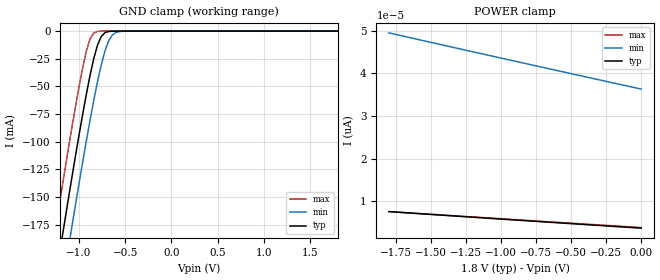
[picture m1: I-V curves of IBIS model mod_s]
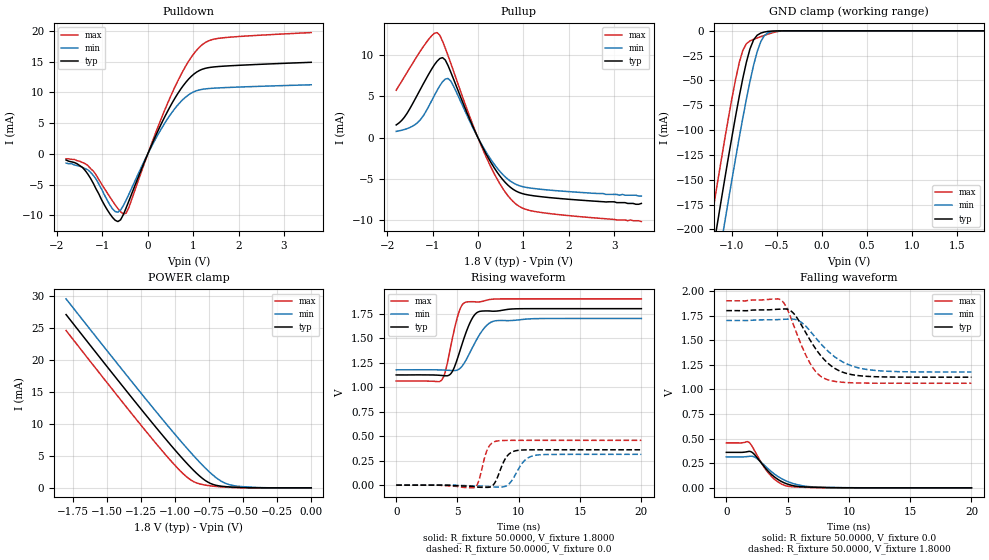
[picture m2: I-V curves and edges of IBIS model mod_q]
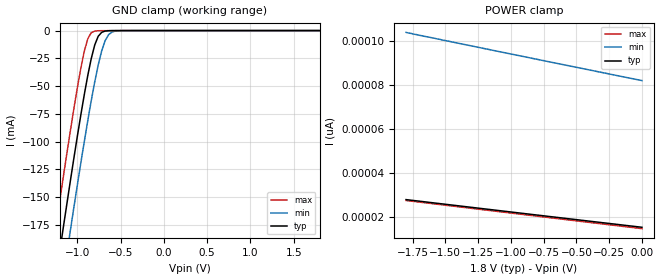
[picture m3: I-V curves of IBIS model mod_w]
| IBIS (I/O, Buffer, Information, Specification) Model, officially
| electronic behavioral standard for Buffer structures of digital pins.
[IBIS ver]  4.0
[File name] m95xxx_tssop8_1d8v.ibs
[File Rev]  16
[Date]  13 December 2012
[Notes]
  (Note1)  This IBIS model includes the TSSOP8 package parasitic data
  (Note2)  This IBIS model considers: VCC= 1.80(TYP), 1.70(MIN), 1.90(MAX)
  (Note3)  This IBIS model has some Notes about the non-monotonicity
   of the I-V curves, but they are not indicative of problems
   inside the model;
[Copyright] (c) 2012 STMicroelectronics
| - M95xxx EEPROM (F8H/P2 process)
| - Voltage Supply Range: 1.7V/1.9V
| - Package: TSSOP8
[Component] M95XXX
[Manufacturer] STMicroelectronics
[Package]
| variable   typ   min   max
R_pkg   0.0   0.0   0.0
L_pkg   0.0H   0.0H   0.0H
C_pkg   0.0F   0.0F   0.0F
[Pin]   signal_name   model_name   R_pin   L_pin   C_pin
1   SN   mod_s   NA   NA   NA
2   Q   mod_q   NA   NA   NA
3   WN   mod_w   NA   NA   NA
4   GND   GND   NA   NA   NA
5   D   mod_s   NA   NA   NA
6   C   mod_s   NA   NA   NA
7   HOLDN   mod_h   NA   NA   NA
8   VCC   POWER   NA   NA   NA
[Package Model]  182696_TSSOP8
[Define Package Model]  182696_TSSOP8
[Manufacturer]  STMicroelectronics
[OEM]  STMicroelectronics
[Description]  8 pin TSSOP package
[Number Of Pins]  8
[Pin Numbers]
|Pin Num   Terminal Name
1   | net1
2   | net2
3   | net3
4   | net4_GND
5   | net5
6   | net6
7   | net7
8   | net8_VDD
[Model Data]
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[End Model Data]
[End Package Model]
| Models and submodels in the file (4): mod_s (Input), mod_q (I/O), mod_w (Input), mod_h (Input)
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|   Model mod_s
[Model]   mod_s   | associated to PIN1 (S), PIN5 (D), PIN6 (CK)
Model_type Input
Vinl   =   0.45V
Vinh   =   1.35V
C_comp   2.119pF   2.023pF   2.433pF
[Temperature Range]   25.0000   85.0000   -40.0000
[Voltage Range]   1.8000V   1.7000V   1.9000V
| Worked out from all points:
|   GND clamp passes 1 mA (typ) near -0.70 V on its own axis
[GND_clamp]
|Voltage   I(typ)   I(min)   I(max)
-1.8V     -520.5mA   -564.7mA   -476.1mA
-1.28V    -238.3mA   -283.2mA   -192.7mA
-1.24V    -217.2mA   -262.1mA   -171.5mA
-1.16V    -175.3mA   -220.1mA   -129.7mA
-1.08V    -134.2mA   -178.7mA   -89.03mA
-920mV    -57.12mA   -99.32mA   -18.15mA
-840mV    -24.96mA   -62.76mA   -1.769mA
-800mV    -12.85mA   -46.02mA   -321.2uA
-720mV    -1.515mA   -18.31mA   -8.596uA
-680mV    -390.8uA   -9.065mA   -1.39uA
-600mV    -23.11uA   -1.27mA    -36.27nA
1.8V      3.691pA    37.05pA    3.633pA
[POWER_clamp]
|Voltage   I(typ)   I(min)   I(max)
-1.8V     7.58pA     49.51pA    7.572pA
-940mV    5.692pA    43.16pA    5.773pA
-440mV    4.62pA     39.51pA    4.74pA
0V        3.691pA    36.33pA    3.838pA
|   Model mod_q
[Model]   mod_q
Model_type I/O
Enable   Active-Low
Vinl   =   0.45V
Vinh   =   1.35V
Vmeas  =   0.9V
Cref   =   30pF
C_comp   3.207pF   2.925pF   3.517pF
[Temperature Range]   25.0000   85.0000   -40.0000
[Voltage Range]   1.8000V   1.7000V   1.9000V
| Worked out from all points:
|   slope of the pulldown table from 0 to 0.27 V, typ, clamps not added: 60.4 ohm
|   slope of the pullup table from 0 to 0.27 V, typ, clamps not added: 94.3 ohm
|   GND clamp passes 1 mA (typ) near -0.63 V on its own axis
|   POWER clamp passes 1 mA (typ) near -0.77 V on its own axis
|   rising waveform, R_fixture 50.0000, V_fixture 1.8000: 20-80 % time 1.14ns typ, 1.42ns min, 892ps max; typ from 1.12 V to 1.8 V
|   rising waveform, R_fixture 50.0000, V_fixture 0.0: 20-80 % time 765ps typ, 960ps min, 603ps max; typ from 0 V to 0.36 V
|   falling waveform, R_fixture 50.0000, V_fixture 0.0: 20-80 % time 1.76ns typ, 2.11ns min, 1.53ns max; typ from 0.36 V to 0 V
|   falling waveform, R_fixture 50.0000, V_fixture 1.8000: 20-80 % time 2.28ns typ, 2.65ns min, 1.76ns max; typ from 1.8 V to 1.12 V
[Pulldown]
|Voltage   I(typ)   I(min)   I(max)
-1.8V     -1mA       -1.5mA     -800uA
-1.44V    -2.2mA     -2.2mA     -1.4mA
-1.26V    -4mA       -3mA       -2.4mA
-720mV    -10.8mA    -9.373mA   -8.283mA
-600mV    -10.73mA   -9.15mA    -9.408mA
-480mV    -8.845mA   -7.565mA   -9.667mA
60mV      1.038mA    875.8uA    1.209mA
420mV     6.704mA    5.539mA    7.96mA
780mV     11.1mA     8.888mA    13.56mA
1.14V     13.58mA    10.42mA    17.38mA
1.56V     14.22mA    10.73mA    18.8mA
3.6V      14.9mA     11.24mA    19.74mA
[Pullup]
|Voltage   I(typ)   I(min)   I(max)
-1.8V     1.541mA    755uA      5.759mA
-1.62V    2.478mA    984uA      7.386mA
-1.32V    5.333mA    1.872mA    10.08mA
-1.02V    8.318mA    4.472mA    12.37mA
-900mV    9.282mA    5.725mA    12.76mA
-780mV    9.719mA    6.785mA    11.73mA
-600mV    7.983mA    6.891mA    9.069mA
120mV     -1.347mA   -1.194mA   -1.582mA
480mV     -4.639mA   -4.079mA   -5.585mA
780mV     -6.301mA   -5.512mA   -7.794mA
1.32V     -7.134mA   -6.241mA   -9.037mA
3.6V      -8mA       -7.1mA     -10.2mA
[GND_clamp]
|Voltage   I(typ)   I(min)   I(max)
-1.8V     -560mA     -602.9mA   -520.9mA
-1.24V    -237mA     -280.8mA   -196.5mA
-1.16V    -192.3mA   -236.1mA   -151.9mA
-1.08V    -148.5mA   -192.1mA   -108.4mA
-960mV    -85.65mA   -128.1mA   -48.54mA
-880mV    -47.76mA   -87.61mA   -19.64mA
-800mV    -18.02mA   -50.66mA   -10.12mA
-760mV    -9.035mA   -34.5mA    -8.516mA
-720mV    -4.395mA   -20.89mA   -7.15mA
-640mV    -1.177mA   -4.777mA   -4.574mA
-520mV    -129.5uA   -385.9uA   -1.208mA
1.8V      141.6pA    24.61nA    124.5pA
[POWER_clamp]
|Voltage   I(typ)   I(min)   I(max)
-1.8V     27.04mA    29.5mA     24.55mA
-1.38V    15.74mA    18.22mA    13.22mA
-1.14V    9.437mA    11.92mA    6.935mA
-980mV    5.408mA    7.841mA    3.048mA
-880mV    3.078mA    5.401mA    1.172mA
-800mV    1.495mA    3.57mA     516.6uA
-740mV    688.2uA    2.33mA     311.5uA
-660mV    257.8uA    1.032mA    143.9uA
-600mV    143uA      487.9uA    68.21uA
-520mV    59.14uA    213.8uA    18.45uA
-380mV    3.968uA    49.9uA     230.5nA
0V        141.6pA    464.6pA    144.1pA
[Ramp]
| variable   typ   min   max
dV/dt_r  0.2164/0.8782n   0.1882/1.1464n   0.2739/0.6586n
dV/dt_f  0.4057/2.4641n   0.3145/2.9896n   0.5034/1.8873n
R_load = 50.0000
[Rising Waveform]
R_fixture= 50.0000
V_fixture= 1.8000
V_fixture_min= 1.7000
V_fixture_max= 1.9000
|time   V(typ)   V(min)   V(max)
0s        1.124V     1.176V     1.062V
3.7ns     1.119V     1.175V     1.069V
4.02ns    1.115V     1.173V     1.164V
4.58ns    1.16V      1.169V     1.496V
5.18ns    1.362V     1.188V     1.786V
5.66ns    1.544V     1.268V     1.865V
6.52ns    1.753V     1.475V     1.868V
7.34ns    1.777V     1.624V     1.885V
7.94ns    1.774V     1.672V     1.898V
20ns      1.8V       1.7V       1.9V
[Rising Waveform]
R_fixture= 50.0000
V_fixture= 0.0
V_fixture_min= 0.0
V_fixture_max= 0.0
|time   V(typ)   V(min)   V(max)
0s        5.912nV    48.36nV    5.653nV
6.42ns    -16.31mV   -8.053mV   -23.14mV
6.72ns    -21.39mV   -8.88mV    39.22mV
7.48ns    -22.74mV   -13.32mV   374.6mV
8.24ns    73.4mV     -20.46mV   450.3mV
9ns       288.3mV    -6.26mV    456.2mV
9.8ns     351.7mV    124.8mV    456.7mV
10.48ns   359mV      251.6mV    456.8mV
11.32ns   360.3mV    303.6mV    456.8mV
20ns      360.5mV    313.9mV    456.8mV
[Falling Waveform]
R_fixture= 50.0000
V_fixture= 0.0
V_fixture_min= 0.0
V_fixture_max= 0.0
|time   V(typ)   V(min)   V(max)
0s        360.5mV    313.9mV    456.8mV
1.84ns    370.1mV    319.5mV    463.2mV
2.4ns     323.3mV    305.7mV    355.7mV
3ns       229.8mV    241.3mV    225.3mV
3.48ns    160.8mV    186mV      144.6mV
4.12ns    93.15mV    122.5mV    68.09mV
4.92ns    41.1mV     68.07mV    18.79mV
6.12ns    11.36mV    23.04mV    6.504mV
7.52ns    4.437mV    7.614mV    1.856mV
20ns      127.1nV    1.308uV    6.709nV
[Falling Waveform]
R_fixture= 50.0000
V_fixture= 1.8000
V_fixture_min= 1.7000
V_fixture_max= 1.9000
|time   V(typ)   V(min)   V(max)
0s        1.8V       1.7V       1.9V
4.44ns    1.815V     1.711V     1.91V
4.9ns     1.816V     1.713V     1.834V
5.46ns    1.775V     1.713V     1.662V
6.86ns    1.496V     1.589V     1.259V
7.54ns    1.369V     1.487V     1.149V
8.3ns     1.264V     1.387V     1.097V
9.7ns     1.166V     1.266V     1.07V
11.52ns   1.132V     1.201V     1.064V
20ns      1.124V     1.176V     1.062V
|   Model mod_w
[Model]   mod_w
Model_type Input
Vinl   =   0.45V
Vinh   =   1.35V
C_comp   2.119pF   2.023pF   2.433pF
[Temperature Range]   25.0000   85.0000   -40.0000
[Voltage Range]   1.8000V   1.7000V   1.9000V
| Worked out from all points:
|   GND clamp passes 1 mA (typ) near -0.70 V on its own axis
[GND_clamp]
|Voltage   I(typ)   I(min)   I(max)
-1.8V     -520.9mA   -565mA     -476.5mA
-1.28V    -238.6mA   -283.5mA   -193mA
-1.24V    -217.4mA   -262.3mA   -171.8mA
-1.16V    -175.4mA   -220.3mA   -129.9mA
-1.08V    -134.3mA   -178.9mA   -89.23mA
-920mV    -57.23mA   -99.42mA   -18.3mA
-840mV    -25.05mA   -62.84mA   -1.898mA
-800mV    -12.93mA   -46.09mA   -437.7uA
-720mV    -1.572mA   -18.35mA   -100.4uA
-680mV    -437uA     -9.101mA   -81.04uA
-600mV    -49.15uA   -1.291mA   -55.89uA
1.8V      15.18pA    83.01pA    13.84pA
[POWER_clamp]
|Voltage   I(typ)   I(min)   I(max)
-1.8V     27.74pA    103.7pA    27.34pA
-1.66V    26.75pA    101.9pA    26.34pA
-1.62V    26.47pA    101.5pA    26.05pA
-1.52V    25.77pA    100.2pA    25.34pA
0V        15.18pA    81.81pA    14.55pA
